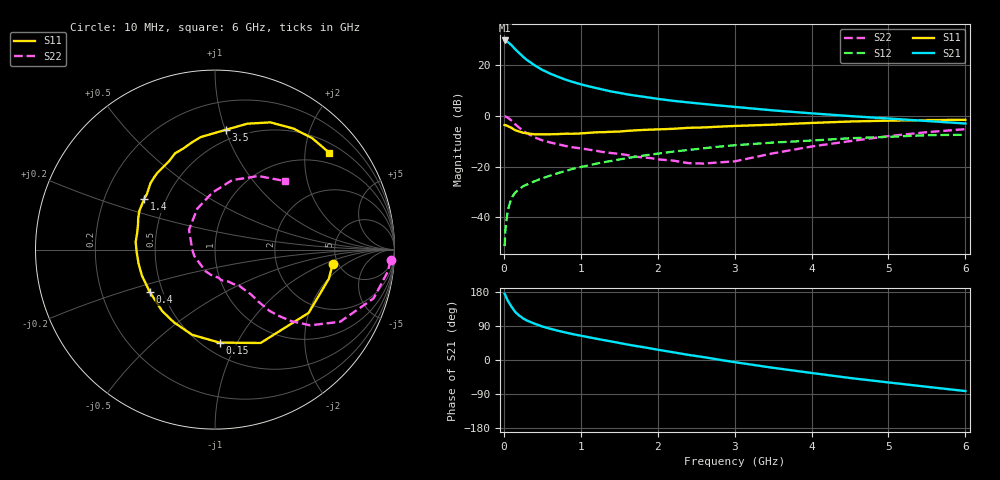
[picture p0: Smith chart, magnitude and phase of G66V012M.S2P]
! SIEMENS Small Signal Semiconductors
! BFG193
! Si NPN RF Bipolar Junction Transistor in SOT223
! VCE = 6 V  IC = 12 mA
! Common Emitter S-Parameters:  August  1996
# GHz  S  MA  R  50
!  f  S11  S21  S12  S22
! GHz  MAG  ANG  MAG  ANG  MAG  ANG  MAG  ANG
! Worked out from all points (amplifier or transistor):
!   36 points, 10 MHz to 6 GHz, reference 50 ohm
!   highest |S21| = 29.7 dB at 10 MHz (marker M1)
!   |S21| within 3 dB of that: start of sweep to 134.1 MHz
!   unconditionally stable (mu >= 1): 860.6 MHz to 2.437 GHz
!   at 250 MHz: K = 0.58, MSG = 25.5 dB, |S12| = -27.7 dB
!   at 1.4 GHz: K = 1.06, MAG = 12.2 dB, |S12| = -17.8 dB
!   at 6 GHz: K = 0.87, MSG = 2.2 dB, |S12| = -7.5 dB
!   S11 on the Smith chart (normalised r, x): 10 MHz: 4.50, -1.30; 150 MHz: 0.60, -0.85; 400 MHz: 0.42, -0.24; 1.4 GHz: 0.38, +0.28; 3.5 GHz: 0.41, +1.00; 6 GHz: 0.71, +2.54
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0.01  0.6605 -7.1  30.59 174.9  0.0027 87.5  0.9798 -3.5
0.02  0.6547 -14.4  30.27 171.0  0.0057 83.9  0.9708 -7.2
0.05  0.6298 -34.0  28.73 157.1  0.0136 75.0  0.9244 -17.1
0.1  0.579 -64.0  24.66 140.5  0.0242 65.2  0.8045 -30.0
0.15  0.5188 -87.2  20.38 126.3  0.0312 58.0  0.6777 -38.5
0.2  0.4915 -105.0  17.24 117.3  0.0357 55.3  0.584 -43.1
0.25  0.4653 -119.5  14.61 109.9  0.041 53.2  0.5062 -46.4
0.3  0.4514 -130.8  12.65 104.2  0.0442 53.0  0.4546 -48.4
0.4  0.4331 -147.2  9.911 95.8  0.0514 53.1  0.3761 -50.2
0.5  0.4323 -160.7  8.042 88.4  0.0588 53.3  0.3287 -51.0
0.6  0.4331 -169.9  6.822 82.7  0.0663 54.0  0.2994 -52.1
0.7  0.4367 -178.2  5.909 77.4  0.074 53.8  0.2759 -53.8
0.9  0.4433 168.3  4.635 68.1  0.0905 53.2  0.2395 -56.3
1.1  0.4618 157.9  3.826 60.2  0.1056 51.9  0.2164 -62.2
1.4  0.4853 144.3  3.013 48.8  0.1294 48.1  0.1845 -71.5
1.7  0.5161 134.1  2.516 37.5  0.1552 43.8  0.1574 -83.1
2.2  0.555 117.5  1.976 20.4  0.1969 34.5  0.1312 -113.7
2.8  0.6124 101.8  1.599 0.8  0.2473 22.5  0.121 -163.7
3.5  0.6701 84.9  1.28 -20.6  0.2971 6.4  0.1825 142.5
4.5  0.773 66.5  0.989 -47.5  0.3618 -13.4  0.3174 92.7
5.5  0.8239 48.9  0.791 -70.7  0.4158 -37.4  0.4764 59.4
6  0.8343 40.4  0.706 -82.0  0.4239 -51.4  0.5468 44.2
